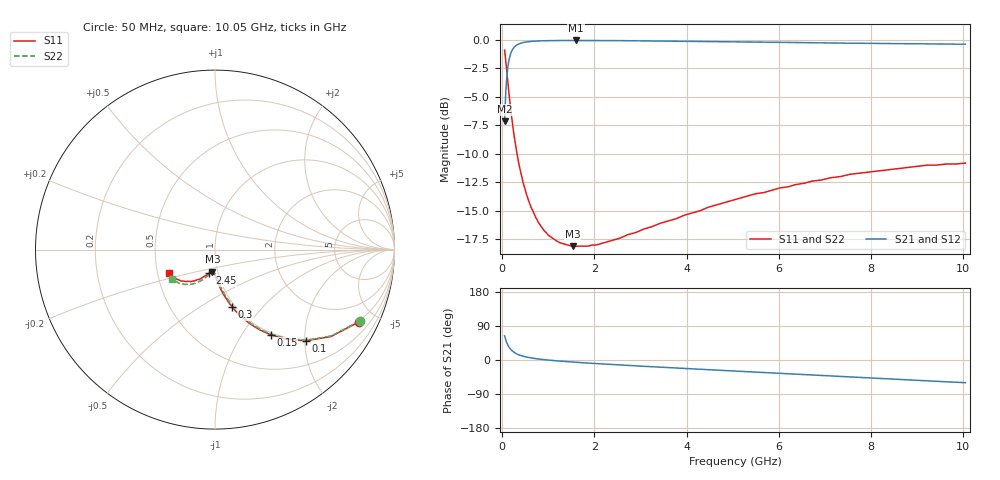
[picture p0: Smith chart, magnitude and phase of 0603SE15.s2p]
! AVX Thin Film Operation		Date: August 2001
! Description: Accu-P® Series, Thin Film, SMD, RF Capacitor
! Part Number: 06033J150FBT
! 50 MHz  -  10.05 GHz
! Serial Measurements
# mhz S db R 50
!	S11		S21		S12		S22
!	dB	Phase	dB	Phase	dB	Phase	dB	Phase
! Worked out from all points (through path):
!   401 points, 50 MHz to 10.05 GHz, reference 50 ohm
!   highest |S21| = -0.07 dB at 1.6 GHz (marker M1); lowest = -7.2 dB at 50 MHz (marker M2)
!   group delay of S21, straight-line fit = 19.7 ps
!   lowest |S11| = -18.1 dB at 1.525 GHz (marker M3), VSWR 1.28, Z = 47.2 - j11.8 ohm
!   |S11| at or under -10 dB: 319.3 MHz to end of sweep
!   |S22| runs from -18.1 to -0.9 dB; largest |S21 - S12| = 0.00011
!   S11 on the Smith chart (normalised r, x): 50 MHz: 0.97, -4.03; 100 MHz: 0.97, -2.02; 150 MHz: 0.97, -1.35; 300 MHz: 0.97, -0.69; 2.45 GHz: 0.91, -0.24; 10.05 GHz: 0.57, -0.16
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50  -0.93 -26.5  -7.17 63.6  -7.17 63.6  -0.93 -26.3
75  -1.86 -36.9  -4.59 53.2  -4.59 53.2  -1.86 -36.6
100  -2.90 -45.2  -3.14 45.0  -3.14 45.0  -2.90 -44.9
125  -3.94 -51.7  -2.25 38.5  -2.25 38.5  -3.94 -51.3
150  -4.94 -56.9  -1.69 33.3  -1.69 33.3  -4.94 -56.5
175  -5.84 -61.0  -1.31 29.2  -1.31 29.2  -5.84 -60.5
225  -7.51 -67.2  -0.85 23.1  -0.85 23.1  -7.51 -66.5
300  -9.55 -73.4  -0.52 17.0  -0.52 17.0  -9.55 -72.5
400  -11.63 -78.6  -0.31 11.9  -0.31 11.9  -11.63 -77.4
500  -13.19 -82.1  -0.22 8.5  -0.22 8.5  -13.19 -80.7
600  -14.43 -84.7  -0.16 6.0  -0.16 6.0  -14.43 -83.0
775  -15.96 -87.9  -0.12 2.8  -0.12 2.8  -15.96 -86.0
1050  -17.27 -91.7  -0.09 -0.8  -0.09 -0.8  -17.27 -89.3
1525  -18.10 -96.5  -0.07 -5.4  -0.07 -5.4  -18.10 -93.6
1600  -18.10 -97.1  -0.07 -6.0  -0.07 -6.0  -18.10 -94.2
1725  -18.10 -98.2  -0.07 -7.0  -0.07 -7.0  -18.10 -95.2
2450  -17.51 -103.9  -0.09 -12.4  -0.09 -12.4  -17.51 -100.0
3400  -16.13 -109.9  -0.12 -18.8  -0.12 -18.8  -16.13 -106.9
5050  -14.02 -121.4  -0.19 -29.3  -0.19 -29.3  -14.02 -116.4
6725  -12.40 -132.0  -0.27 -39.5  -0.27 -39.5  -12.39 -126.0
8400  -11.39 -143.1  -0.35 -49.8  -0.35 -49.8  -11.29 -136.1
10050  -10.82 -153.6  -0.40 -59.9  -0.40 -59.9  -10.80 -145.8
